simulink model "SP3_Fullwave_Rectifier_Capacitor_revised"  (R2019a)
settings: Solver=VariableStepAuto  StartTime=0  StopTime=0.05  FixedStep=1e-5  RelTol=1e-6
libraries: fl_lib x9, nesl_utility x5

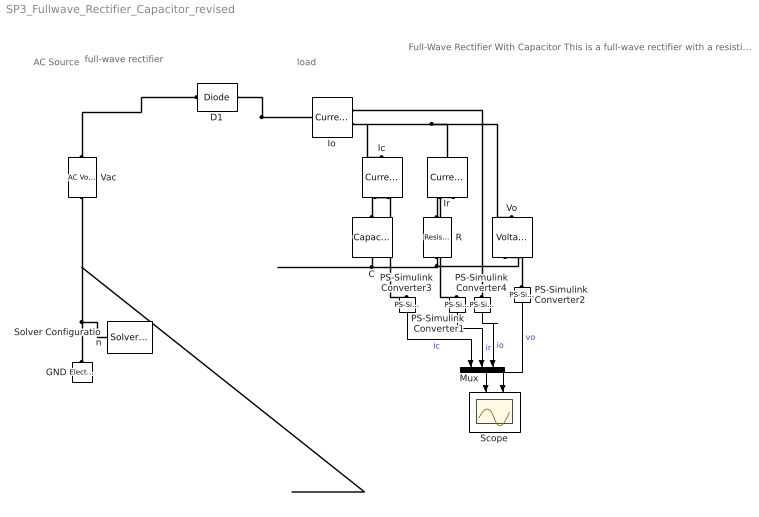
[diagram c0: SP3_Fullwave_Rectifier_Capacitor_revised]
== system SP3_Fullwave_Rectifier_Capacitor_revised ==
  note: Full-Wave Rectifier With Capacitor This is a full-wave rectifier with a resistive and parallel capacitor load. 1. One ideal diode is placed, but the other three need to be added. Copy and paste the existing diode. 2. Place the other three diodes to make the full-wave rectifier. Press Ctrl+R to rotate a component. C1. Capture the complete circuit diagram. 3. Simulate the circuit (click the Run button above). 4. Open the Scope below (double click). 5. Observe the current and voltage waveforms. C2. Capture the three current (top plot) and one voltage (bottom plot) waveforms. 6. In the scope, see that "Signal Statistics" give the maximum and minimum values. 7. Above "Signal Statistics," you can select different signals to see their values. Q1. What is the output voltage ripple? Q2. What is maximum output current (Io) value? ------------------------------------------------------- The maximum output current value is too high for your design specification. 8. Go back to the "Simulink" window. 9. Double click on capacitor C to see it's properties. 10. Determine the value of capacitor C so that the maximum output current is approximately 15 A. 11. Click on the "Run" button on the top bar or press "CTRL + T". C3. Capture the new current and voltage waveforms. Q3. What is the new capacitor value? Q4. What is the new output voltage ripple? Q5. Explain how the capacitor value affects output voltage ripple and current spikes. _________________________________ Play: Try changing the capacitor and resistor values. Observe how the shape of the current and voltage waveforms change.
  note: load
  note: AC Source
  note: full-wave rectifier
  C : fl_lib/Electrical/Electrical Elements/Capacitor  c=2200 uF  r=1e-6 Ohm  g=0 1/Ohm  i_specify=off  i_priority=None  i=0 A  i_nominal_specify=off  i_nominal_unit=A  i_nominal_value=1  v_specify=off  v_priority=None  v=0 V  v_nominal_specify=off  v_nominal_unit=V  v_nominal_value=1  vc_specify=off  vc_priority=High  vc=0 V  vc_nominal_specify=off  vc_nominal_unit=V  vc_nominal_value=1
  D1 : fl_lib/Electrical/Electrical Elements/Diode  Vf=1e-3 V  Ron=1e-3 Ohm  Goff=1e-8 1/Ohm  i_specify=off  i_priority=None  i=0 A  i_nominal_specify=off  i_nominal_unit=A  i_nominal_value=1  v_specify=off  v_priority=None  v=0 V  v_nominal_specify=off  v_nominal_unit=V  v_nominal_value=1
  GND : fl_lib/Electrical/Electrical Elements/Electrical Reference
  Ic : fl_lib/Electrical/Electrical Sensors/Current Sensor
  Io : fl_lib/Electrical/Electrical Sensors/Current Sensor
  Ir : fl_lib/Electrical/Electrical Sensors/Current Sensor
  Mux : Mux  Inputs=3
  PS-Simulink Converter{1..4} (4 alike) : nesl_utility/PS-Simulink Converter  PhysicalDomain=network_engine_domain  SubClassName=ps_output  LeftPortType=input  RightPortType=output  PseudoPeriodic=off  Frequencies=[]  Unit=1  AffineConversion=off
  R : fl_lib/Electrical/Electrical Elements/Resistor  R=100 Ohm  i_specify=off  i_priority=None  i=0 A  i_nominal_specify=off  i_nominal_unit=A  i_nominal_value=1  v_specify=off  v_priority=None  v=0 V  v_nominal_specify=off  v_nominal_unit=V  v_nominal_value=1
  Scope : Scope  NumInputPorts=2
  Solver Configuration : nesl_utility/Solver Configuration  PhysicalDomain=network_engine_domain  SubClassName=solver  LeftPortType=input  RightPortType=generic  Tones=[]  Harmonics=[]  SimulateNoise=off  Profile=off  UseLocalSampling=off  EnableSwitchedLinearOptims=on  FrequencyDomain=off  UseCCode=off  RelTol=0.001  AbsTol=1e-06  MinStep=1e-09  ToWorkspace=off  RevertToSquareIcSolve=off  NumHomotopyIterations=100  PhasorMode=off  PhasorModeNumHarmonics=1  DoDC=off  ResidualTolerance=1e-09  UseLocalSolver=off  LocalSolverChoice=NE_BACKWARD_EULER_ADVANCER  LocalSolverSampleTime=0.001  DoFixedCost=off  MaxNonlinIter=3  MaxModeIter=2  LinearAlgebra=auto  EquationFormulation=NE_TIME_EF  DelaysMemoryBudget=1024  AutomaticFiltering=on  FilteringTimeConstant=0.001  PartitionStorageMethod=AS_NEEDED  PartitionMemoryBudget=1024  PartitionMethod=ROBUST
  Vac : fl_lib/Electrical/Electrical Sources/AC Voltage Source  amp=311 V  shift=0 deg  frequency=60 Hz  omega=0 rad/s
  Vo : fl_lib/Electrical/Electrical Sensors/Voltage Sensor
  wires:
  Mux/1 -> Scope/1
  PS-Simulink Converter2/1 -> Scope/2  "vo"
  PS-Simulink Converter4/1 -> Mux/3  "io"
  PS-Simulink Converter1/1 -> Mux/2  "ir"
  PS-Simulink Converter3/1 -> Mux/1  "ic"
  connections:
  Vac/RConn1 -- Solver Configuration/RConn1 -- GND/LConn1
  Io/RConn2 -- Ir/LConn1 -- Vo/LConn1 -- Ic/LConn1
  PS-Simulink Converter2/LConn1 -- Vo/RConn1
  Ir/RConn1 -- PS-Simulink Converter1/LConn1
  Vac/LConn1 -- D1/LConn1
  D1/RConn1 -- Io/LConn1
  C/LConn1 -- Ic/RConn2
  R/LConn1 -- Ir/RConn2
  R/RConn1 -- Vo/RConn2 -- C/RConn1
  Ic/RConn1 -- PS-Simulink Converter3/LConn1
  PS-Simulink Converter4/LConn1 -- Io/RConn1
